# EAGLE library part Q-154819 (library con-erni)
Male Connector SMC-Q 26 contacts Type 7-13 - Low Profile Source: http://www.erni.com/DB/PDF-Drawing/SMC/154819.pdf
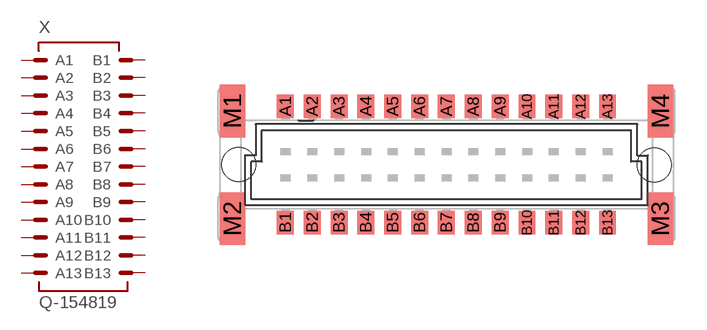
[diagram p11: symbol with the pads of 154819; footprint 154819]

Designator prefix X

## Q-154819 (OC_FARNELL: unknown; OC_NEWARK: unknown)  [154819]
A1  A1  pas
A2  A2  pas
A3  A3  pas
A4  A4  pas
A5  A5  pas
A6  A6  pas
A7  A7  pas
A8  A8  pas
A9  A9  pas
A10  A10  pas
A11  A11  pas
A12  A12  pas
A13  A13  pas
B1  B1  pas
B2  B2  pas
B3  B3  pas
B4  B4  pas
B5  B5  pas
B6  B6  pas
B7  B7  pas
B8  B8  pas
B9  B9  pas
B10  B10  pas
B11  B11  pas
B12  B12  pas
B13  B13  pas

## Footprint 154819 (pad centres in mm)
Male Connector SMC-Q 26 contacts Type 7-13 - Low Profile Source: http://www.erni.com/DB/PDF-Drawing/SMC/154819.pdf
smd 0.8 x 1.1: A1 -7.62,2.765; A2 -6.35,2.765; A3 -5.08,2.765; A4 -3.81,2.765; A5 -2.54,2.765; A6 -1.27,2.765; A7 0,2.765; A8 1.27,2.765; A9 2.54,2.765; A10 3.81,2.765; A11 5.08,2.765; A12 6.35,2.765; A13 7.62,2.765; B1 -7.62,-2.74; B2 -6.35,-2.74; B3 -5.08,-2.74; B4 -3.81,-2.74; B5 -2.54,-2.74; B6 -1.27,-2.74; B7 0,-2.74; B8 1.27,-2.74; B9 2.54,-2.74; B10 3.81,-2.74; B11 5.08,-2.74; B12 6.35,-2.74; B13 7.62,-2.74
smd 1.2 x 2.5: M1 -10.125,2.55; M2 -10.125,-2.55; M3 10.125,-2.55; M4 10.125,2.55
